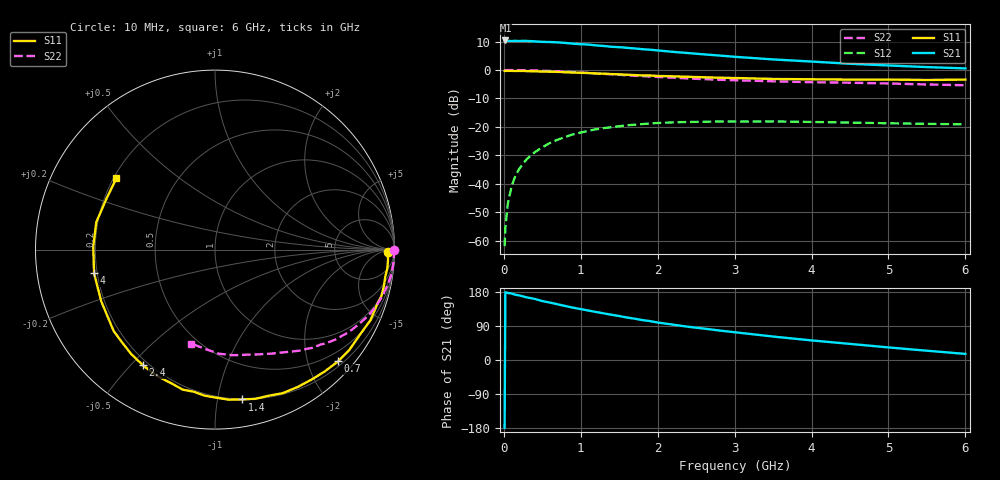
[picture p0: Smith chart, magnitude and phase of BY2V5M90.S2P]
! SIEMENS Small Signal Semiconductors
! BFY420
! Si NPN RF SIEGET Grounded Emitter Transistor in MICRO-X
! VCE = 2.5 V  IC = 0.9 mA
! Common Emitter S-Parameters:  October  1996
# GHz  S  MA  R  50
!  f  S11  S21  S12  S22
! GHz  MAG  ANG  MAG  ANG  MAG  ANG  MAG  ANG
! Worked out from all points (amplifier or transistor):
!   36 points, 10 MHz to 6 GHz, reference 50 ohm
!   highest |S21| = 10.4 dB at 20 MHz (marker M1)
!   |S21| within 3 dB of that: start of sweep to 1.774 GHz
!   unconditionally stable (mu >= 1): 4.566 GHz to end of sweep
!   at 250 MHz: K = 0.03, MSG = 21.6 dB, |S12| = -32.9 dB
!   at 1.4 GHz: K = 0.19, MSG = 14.1 dB, |S12| = -20.1 dB
!   at 6 GHz: K = 1.36, MAG = 6.3 dB, |S12| = -19.1 dB
!   S11 on the Smith chart (normalised r, x): 10 MHz: 48, -19; 700 MHz: 0.29, -2.56; 1.4 GHz: 0.20, -1.18; 2.4 GHz: 0.18, -0.54; 4 GHz: 0.19, -0.09; 6 GHz: 0.21, +0.31
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0.01  0.9645 -0.8  3.296 -179.4  0.0008 98.8  0.9989 -0.2
0.02  0.9612 -1.2  3.307 178.8  0.0017 100.3  0.9922 -0.5
0.05  0.9658 -3.3  3.244 177.0  0.0043 88.3  0.9973 -1.4
0.1  0.966 -6.3  3.239 175.6  0.009 86.6  0.9972 -3.0
0.15  0.9606 -9.0  3.244 172.1  0.0138 82.9  0.9961 -4.4
0.2  0.9629 -12.5  3.234 170.4  0.0182 82.9  0.995 -5.8
0.3  0.954 -18.3  3.242 165.2  0.0272 79.1  0.9898 -8.8
0.4  0.9512 -24.4  3.19 161.3  0.0357 75.1  0.9817 -11.7
0.5  0.9363 -30.4  3.123 155.5  0.0438 71.4  0.9712 -14.5
0.7  0.9264 -42.2  3.059 147.0  0.0596 64.6  0.947 -20.0
0.9  0.9019 -53.5  2.9 138.0  0.0739 57.3  0.9175 -25.1
1.1  0.8846 -64.7  2.8 130.4  0.0856 51.1  0.8865 -29.9
1.4  0.8483 -79.8  2.559 119.4  0.0986 42.6  0.8407 -36.4
1.8  0.8003 -98.6  2.324 105.3  0.112 32.6  0.7802 -43.6
2.2  0.7745 -114.9  2.083 93.3  0.1201 24.3  0.7334 -50.2
2.4  0.7593 -121.9  1.983 87.6  0.1221 20.9  0.7094 -53.2
2.8  0.7313 -135.3  1.797 77.8  0.1246 14.8  0.6739 -58.6
3.5  0.6962 -155.6  1.535 61.9  0.1246 6.8  0.6327 -67.3
4  0.6866 -168.9  1.408 51.7  0.1223 2.7  0.6105 -73.6
4.5  0.6785 178.7  1.287 42.5  0.119 -0.6  0.5973 -80.2
5.5  0.668 155.0  1.125 24.5  0.1132 -2.9  0.5564 -95.6
6  0.6778 144.2  1.067 16.0  0.1105 -2.3  0.5398 -104.2
